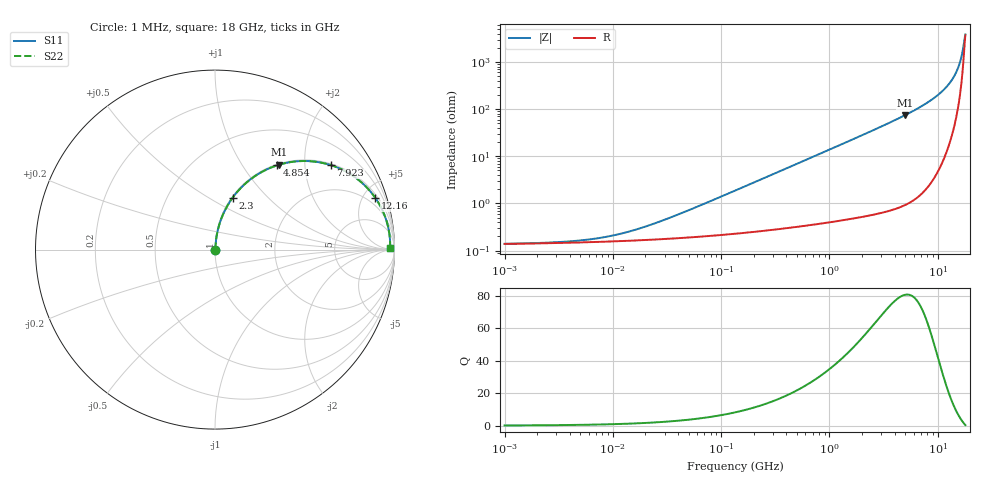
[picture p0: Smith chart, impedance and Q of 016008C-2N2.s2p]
# MHz S MA R 50
!Freq  MagS11  AngS11  MagS21  AngS21  MagS12  AngS12  MagS22  AngS22
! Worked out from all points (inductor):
!   801 points, 1 MHz to 18 GHz, reference 50 ohm
!   read as one part in series: L = 2.2 nH near 39.91 MHz
!   highest Q = 80.7 at 4.975 GHz (marker M1), where L = 2.38 nH
!   S11 on the Smith chart (normalised r, x): 1 MHz: 1.00, +0.00; 2.3 GHz: 1.01, +0.65; 4.854 GHz: 1.02, +1.45; 7.923 GHz: 1.04, +2.71; 12.16 GHz: 1.26, +6.09; 18 GHz: 75, +22
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1  0.001389 5.7  0.9986 -0.0  0.9986 -0.0  0.001389 5.7
2.631529  0.001479 14.2  0.9986 -0.0  0.9986 -0.0  0.001479 14.2
5.161289  0.00165 25.5  0.9985 -0.0  0.9985 -0.0  0.00165 25.5
11.58292  0.00225 45.2  0.9984 -0.1  0.9984 -0.1  0.00225 45.2
26.31463  0.004021 64.3  0.9983 -0.2  0.9983 -0.2  0.004021 64.3
134.1641  0.01864 82.0  0.9976 -1.1  0.9976 -1.1  0.01864 82.0
340.3197  0.04696 83.8  0.9961 -2.7  0.9961 -2.7  0.04696 83.8
692.4595  0.09515 82.4  0.992 -5.5  0.992 -5.5  0.09515 82.4
1293.207  0.1762 78.5  0.9801 -10.1  0.9801 -10.1  0.1762 78.5
2299.669  0.3059 71.2  0.9469 -17.8  0.9469 -17.8  0.3059 71.2
3530.478  0.4499 62.5  0.8869 -26.7  0.8869 -26.7  0.4499 62.5
4854.336  0.5824 53.7  0.8057 -35.6  0.8057 -35.6  0.5824 53.7
4974.713  0.5932 52.9  0.7977 -36.4  0.7977 -36.4  0.5932 52.9
6355.501  0.7031 44.6  0.7021 -44.7  0.7021 -44.7  0.7031 44.6
7923.069  0.7984 36.1  0.59 -53.0  0.59 -53.0  0.7984 36.1
9998.99  0.8847 26.5  0.4458 -62.2  0.4458 -62.2  0.8847 26.5
12163.59  0.9384 17.9  0.3078 -69.6  0.3078 -69.6  0.9384 17.9
13917.83  0.9625 11.9  0.2069 -73.7  0.2069 -73.7  0.9625 11.9
15350.56  0.9728 7.5  0.1322 -74.4  0.1322 -74.4  0.9728 7.5
16319.99  0.9759 4.8  0.08584 -71.3  0.08584 -71.3  0.9759 4.8
17350.63  0.9765 2.0  0.04241 -55.3  0.04241 -55.3  0.9765 2.0
18000  0.9757 0.4  0.02538 -16.1  0.02538 -16.1  0.9757 0.4
